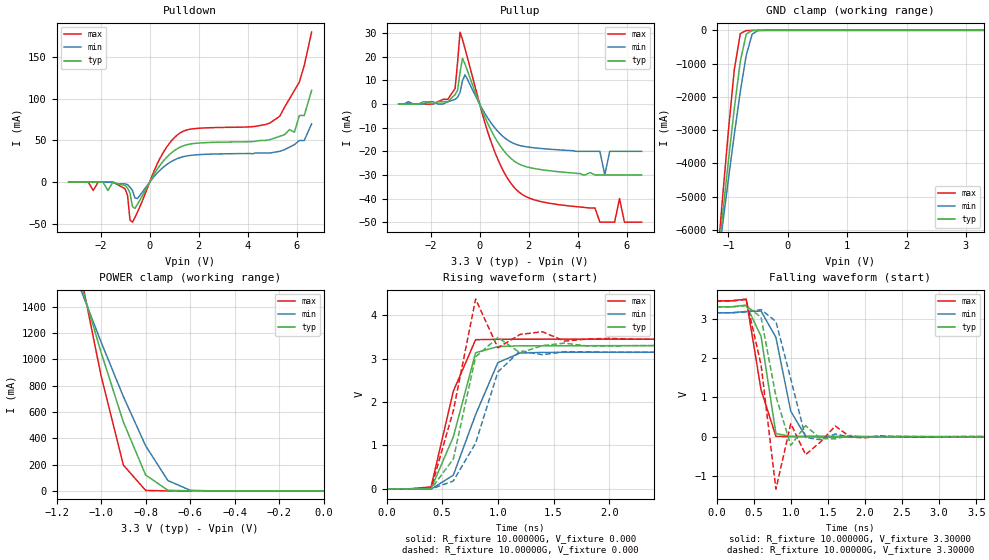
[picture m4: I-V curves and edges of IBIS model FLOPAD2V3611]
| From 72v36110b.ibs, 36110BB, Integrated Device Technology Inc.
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|   Model FLOPAD2V3611
[Model]   FLOPAD2V3611
Model_type   3-state
Polarity   Non-Inverting
Enable   Active-High
Vmeas =  1.50000V
C_comp   10.00000pF   10.00000pF   10.00000pF
[Temperature Range]   25.00000   85.00000   -40.00000
[Voltage Range]   3.30000V   3.15000V   3.45000V
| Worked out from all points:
|   slope of the pulldown table from 0 to 0.495 V, typ, clamps not added: 21.5 ohm
|   slope of the pullup table from 0 to 0.495 V, typ, clamps not added: 42.4 ohm
|   GND clamp passes 1 mA (typ) near -0.52 V on its own axis
|   POWER clamp passes 1 mA (typ) near -0.62 V on its own axis
|   rising waveform, R_fixture 10.00000G, V_fixture 0.000: 20-80 % time 239ps typ, 290ps min, 227ps max; typ from 0 V to 3.3 V
|   rising waveform, R_fixture 10.00000G, V_fixture 0.000: 20-80 % time 174ps typ, 276ps min, 199ps max; typ from 0 V to 3.3 V
|   falling waveform, R_fixture 10.00000G, V_fixture 3.30000: 20-80 % time 175ps typ, 205ps min, 221ps max; typ from 3.3 V to 0 V
|   falling waveform, R_fixture 10.00000G, V_fixture 3.30000: 20-80 % time 220ps typ, 257ps min, 185ps max; typ from 3.3 V to -0.002 V
[Pulldown]
| voltage   I(typ)   I(min)   I(max)
-3.3V     0A         0A         0A
-1V       -4mA       -2mA       -8mA
-800mV    -13.1mA    -6mA       -45.44mA
-700mV    -29.4mA    -10mA      -47.99mA
-500mV    -26.74mA   -19.63mA   -36.09mA
400mV     19.36mA    13.74mA    27.32mA
1.2V      41.38mA    29.07mA    58.2mA
5.3V      55mA       37mA       79mA
5.9V      60mA       45mA       110mA
6.1V      80mA       50mA       120mA
6.3V      80mA       50mA       140mA
6.6V      110mA      70mA       180mA
[Pullup]
| voltage   I(typ)   I(min)   I(max)
-3.3V     0A         0A         0A
-1.3V     1mA        1mA        2mA
-1V       4mA        2mA        6.6mA
-800mV    13.4mA     4.9mA      30.49mA
-600mV    17.05mA    12.41mA    23.59mA
500mV     -11.77mA   -8.469mA   -17mA
1.5V      -24.75mA   -17.12mA   -36.28mA
4.9V      -30mA      -20mA      -50mA
5.1V      -30mA      -30mA      -50mA
5.7V      -30mA      -20mA      -40mA
5.9V      -30mA      -20mA      -50mA
6.6V      -30mA      -20mA      -50mA
[GND_clamp]
| voltage   I(typ)   I(min)   I(max)
-3.3V     -44.86A    -38.5A     -54.32A
-1.2V     -7.292A    -7.294A    -7.196A
-1.1V     -5.587A    -5.872A    -5.069A
-1V       -3.924A    -4.477A    -3.02A
-900mV    -2.338A    -3.123A    -1.172A
-800mV    -940.2mA   -1.846A    -98.36mA
-700mV    -115.7mA   -749mA     -8.05mA
-600mV    -4.278mA   -114.8mA   -2.238mA
-500mV    -295.2uA   -5.816mA   -325.4uA
3.3V      607.7pA    5.602nA    92.72pA
[POWER_clamp]
| voltage   I(typ)   I(min)   I(max)
-3.3V     15.46A     11.9A      22.55A
-1.1V     1.627A     1.567A     1.714A
-1V       1.053A     1.131A     875.2mA
-900mV    523.9mA    716.9mA    196.8mA
-800mV    121.2mA    343.1mA    4.086mA
-700mV    5.031mA    78.95mA    112.4uA
-600mV    111.5uA    5.081mA    8.814uA
0V        607.7pA    2.814nA    110.2pA
[Ramp]
| variable   typ   min   max
dV/dt_r   0.80040/0.24935n   0.55518/0.34835n   1.11420/0.17021n
dV/dt_f   1.24980/0.48363n   0.95160/0.80240n   1.51836/0.26104n
R_load = 50.00000
[Rising Waveform]
R_fixture = 10.00000G
V_fixture = 0.000
V_fixture_min = 0.000
V_fixture_max = 0.000
| time   V(typ)   V(min)   V(max)
0s        0V         0V         0V
200ps     -592.5uV   -37.45uV   -1.019mV
400ps     3.601mV    -8.441mV   43.48mV
600ps     1.197V     314.4mV    2.251V
800ps     3.137V     1.711V     3.438V
1ns       3.28V      2.91V      3.448V
1.2ns     3.298V     3.131V     3.449V
1.8ns     3.299V     3.149V     3.45V
10ns      3.3V       3.15V      3.45V
[Rising Waveform]
R_fixture = 10.00000G
V_fixture = 0.000
V_fixture_min = 0.000
V_fixture_max = 0.000
R_dut = 0.18000
L_dut = 8.10000nH
C_dut = 0.53000pF
| time   V(typ)   V(min)   V(max)
0s        0V         0V         0V
400ps     -4.945mV   -6.345mV   8.207mV
600ps     687.1mV    181.1mV    1.798V
800ps     3.042V     1.053V     4.375V
1ns       3.488V     2.693V     3.251V
1.2ns     3.137V     3.182V     3.56V
1.4ns     3.301V     3.091V     3.622V
1.6ns     3.359V     3.162V     3.405V
1.8ns     3.293V     3.158V     3.453V
10ns      3.298V     3.148V     3.453V
[Falling Waveform]
R_fixture = 10.00000G
V_fixture = 3.30000
V_fixture_min = 3.15000
V_fixture_max = 3.45000
| time   V(typ)   V(min)   V(max)
0s        3.3V       3.15V      3.45V
200ps     3.301V     3.15V      3.453V
400ps     3.345V     3.183V     3.498V
600ps     2.552V     3.192V     1.191V
800ps     79.6mV     2.525V     8.023mV
1ns       8.737mV    647.8mV    3.594mV
1.2ns     4.579mV    12.73mV    1.742mV
10ns      2.865uV    0V         3.049uV
[Falling Waveform]
R_fixture = 10.00000G
V_fixture = 3.30000
V_fixture_min = 3.15000
V_fixture_max = 3.45000
R_dut = 0.18000
L_dut = 8.10000nH
C_dut = 0.53000pF
| time   V(typ)   V(min)   V(max)
0s        3.3V       3.15V      3.45V
400ps     3.328V     3.17V      3.483V
600ps     3.037V     3.229V     1.824V
800ps     1.03V      2.929V     -1.333V
1ns       -219mV     1.468V     329.9mV
1.2ns     281.4mV    -19.9mV    -455.9mV
1.4ns     -48.7mV    -75.4mV    -134.1mV
1.6ns     -53.66mV   68.1mV     271.8mV
2ns       -11.69mV   -19.86mV   -28.17mV
10ns      -1.912mV   -317.7uV   -732.4uV
